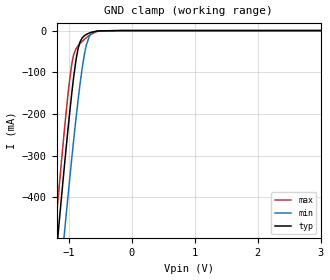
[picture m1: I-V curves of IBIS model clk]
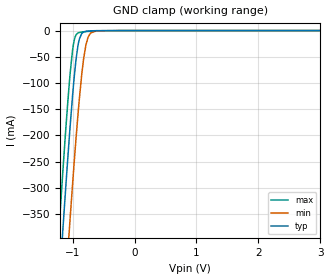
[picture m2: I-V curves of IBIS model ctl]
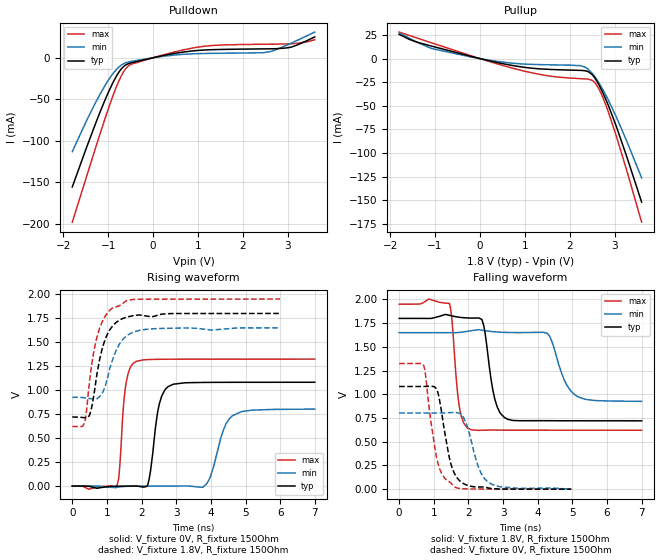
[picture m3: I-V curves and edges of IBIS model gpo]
|Texas Instruments Incorporated
| TPS650860 Configurable Multi-Rail PMIC for 2S & 3S Li-Ion
| Battery-Operated Devices
| Marketing part#   Digital Voltage Range   Package-type   #pins
| TPS650860A0RSKT   1.65V - 1.95V   VQFN   64
[IBIS Ver]   4.1
[File name]   tps650860.ibs
[File Rev]   1.0
[Date]   9/9/2015
[Source]
| Texas Instruments Incorporated.
| Analog-eLab Design Center, HPA
| 12500 TI Blvd
| Dallas, TX -75243
[Notes]   Revision History:
| Rev 1.0: 9/9/2015
| - Initial version of the model
| - Model generated from simulations in TISPICE
| - Model matched to SPICE simulation
| - C_comp although listed in numerical order of value are
|   obtained from varying PVT conditions. For PVT conditions for
|   each specific value refer the buffer description under
|   respective [Model]. IBIS model user is responsible for using
|   appropriate C_comp to simulate for Signal Integrity.
[Disclaimer]
| This model is designed as an aid for customers of Texas Instruments.
| TI and its licensors and suppliers make no warranties, either expressed
| or implied, with respect to this  model, including the warranties of
| merchantability or fitness for a particular purpose. The model is
| provided solely on an "as is" basis. The entire risk as to its quality
| and performance is with the customer.
[Copyright]
(C) Copyright 2014 Texas Instruments Incorporated.All rights reserved.
|   TPS650860A0RSKT
[Component]   TPS650860A0RSKT
[Manufacturer]   TI
[Package]   |64 VQFN  -  RSK package
|   typ   min   max
R_pkg   0.2   0.16   0.24
L_pkg   1.5nH   1.2nH   1.8nH
C_pkg   0.4pF   0.32pF   0.48pF
[Pin]  signal_name   model_name   R_pin   L_pin   C_pin
1   FBGND2   nc   NA   NA   NA
2   FBVOUT2   nc   NA   NA   NA
3   DRVH2   nc   NA   NA   NA
4   SW2   nc   NA   NA   NA
5   BOOT2   nc   NA   NA   NA
6   PGNDSNS2   gnd   NA   NA   NA
7   DRVL2   nc   NA   NA   NA
8   DRV5V_2_A1   power   NA   NA   NA
9   LDOA1   nc   NA   NA   NA
10   LX3   nc   NA   NA   NA
11   PVIN3   power   NA   NA   NA
12   FB3   nc   NA   NA   NA
13   CTL1   ctl   NA   NA   NA
14   CTL6/SLPENB2   ctl   NA   NA   NA
15   IRQB   irqb   NA   NA   NA
16   GPO1   gpox   NA   NA   NA
17   SWB1   nc   NA   NA   NA
18   PVINSWB1_B2   power   NA   NA   NA
19   SWB2   nc   NA   NA   NA
20   LX5   nc   NA   NA   NA
21   PVIN5   power   NA   NA   NA
22   FB5   nc   NA   NA   NA
23   FB4   nc   NA   NA   NA
24   PVIN4   power   NA   NA   NA
25   LX4   nc   NA   NA   NA
26   GPO2   gpox   NA   NA   NA
27   GPO3   gpox   NA   NA   NA
28   GPO4   gpox   NA   NA   NA
29   FBVOUT1   nc   NA   NA   NA
30   ILIM1   nc   NA   NA   NA
31   SWA1   nc   NA   NA   NA
32   PVINSWA1   power   NA   NA   NA
33   DRVH1   nc   NA   NA   NA
34   SW1   nc   NA   NA   NA
35   BOOT1   nc   NA   NA   NA
36   PGNDSNS1   gnd   NA   NA   NA
37   DRVL1   nc   NA   NA   NA
38   DRV5V_1_6   power   NA   NA   NA
39   DRVL6   nc   NA   NA   NA
40   PGNDSNS6   gnd   NA   NA   NA
41   BOOT6   nc   NA   NA   NA
42   SW6   nc   NA   NA   NA
43   DRVH6   nc   NA   NA   NA
44   FBVOUT6   nc   NA   NA   NA
45   ILIM6   nc   NA   NA   NA
46   PVINVTT   power   NA   NA   NA
47   VTT   nc   NA   NA   NA
48   VTTFB   nc   NA   NA   NA
49   LDOA3   nc   NA   NA   NA
50   PVINLDOA2_A3   power   NA   NA   NA
51   LDOA2   nc   NA   NA   NA
52   AGND   gnd   NA   NA   NA
53   VREF   nc   NA   NA   NA
54   LDO3P3   nc   NA   NA   NA
55   VSYS   power   NA   NA   NA
56   LDO5P0   nc   NA   NA   NA
57   V5ANA   power   NA   NA   NA
58   CLK   clk   NA   NA   NA
59   DATA   data   NA   NA   NA
60   CTL2   ctl   NA   NA   NA
61   CTL3/SLPENB1   ctl   NA   NA   NA
62   CTL4   ctl   NA   NA   NA
63   CTL5   ctl   NA   NA   NA
64   ILIM2   nc   NA   NA   NA
|   Model Selectors
[Model Selector] data
data_std   1.8V  digital I/O_Open_drain
data_hs   1.8V  digital I/O_Open_drain
[Model Selector] gpox
gpo   1.8V  digital Output
gpo_od   1.8V  digital Open_drain
| Models and submodels in the file (7): clk (Input), ctl (Input), gpo (Output), gpo_od (Open_drain), data_std (I/O_open_drain), data_hs (I/O_open_drain), irqb (Open_drain)
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|   clk Model
[Model]   clk
Model_type   Input
Vinl = 0.4
Vinh = 1.2
|   typ   min   max
|   (nom PVT)   (fast PVT)   (slow PVT)
C_comp   1.465e-12   1.404e-12   1.531e-12
| Where nom  PVT is Nominal Process, 1.8V, 27C
|   Fast PVT is Strong Process,  1.95V, -40C
|   Slow PVT is Weak Process,   1.65V, 125C
[Voltage Range]   1.8   1.65   1.95
|Junction Temperature
[Temperature Range]   27   125   -40
[Power Clamp Reference]   1.8   1.65   1.95
[GND Clamp Reference]   0   0   0
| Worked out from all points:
|   GND clamp passes 1 mA (typ) near -0.54 V on its own axis
[GND Clamp]
|   Voltage   I(typ)   I(min)   I(max)
-1.8V     -1.585A    -1.712A    -1.529A
-1.417V   -903.9mA   -1.052A    -830.1mA
-1.201V   -532.4mA   -690.5mA   -448.4mA
-1.17V    -480.2mA   -639.5mA   -395mA
-1.076V   -327.4mA   -488.9mA   -240.6mA
-959.6mV  -153.1mA   -309.5mA   -82.58mA
-887.4mV  -67.95mA   -206.8mA   -42.91mA
-828mV    -27.88mA   -130.5mA   -31.56mA
-722.6mV  -8.948mA   -32.89mA   -16.64mA
-648.3mV  -4.138mA   -7.502mA   -8.538mA
-516.9mV  -657.9uA   -778.2uA   -1.114mA
3.6V      0A         0A         0A
[POWER Clamp]
|   Voltage   I(typ)   I(min)   I(max)
-1.8V     0A         0A         0A
0V        0A         0A         0A
3.6V      0A         0A         0A
|   ctl Model
[Model]   ctl
Model_type   Input
Vinl = 0.4
Vinh = 1.2
|   typ   min   max
|   (nom PVT)   (fast PVT)   (slow PVT)
C_comp   4.431e-13   4.006e-13   4.876e-13
| Where nom  PVT is Nominal Process, 1.8V, 27C
|   Fast PVT is Strong Process,  1.95V, -40C
|   Slow PVT is Weak Process,   1.65V, 125C
[Voltage Range]   1.8   1.65   1.95
|Junction Temperature
[Temperature Range]   27   125   -40
[Power Clamp Reference]   1.8   1.65   1.95
[GND Clamp Reference]   0   0   0
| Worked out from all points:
|   GND clamp passes 1 mA (typ) near -0.76 V on its own axis
[GND Clamp]
|   Voltage   I(typ)   I(min)   I(max)
-1.8V     -1.6A      -1.776A    -1.496A
-1.224V   -501.7mA   -684.6mA   -389.4mA
-1.153V   -374.6mA   -556.8mA   -263mA
-1.054V   -206.9mA   -383.9mA   -102.9mA
-986.4mV  -106.2mA   -271.9mA   -26.76mA
-959.6mV  -72.63mA   -229.8mA   -12.55mA
-914.4mV  -30.13mA   -163.2mA   -4.668mA
-851.2mV  -5.575mA   -83.45mA   -2.788mA
-784.8mV  -1.372mA   -27.75mA   -1.943mA
-711mV    -557uA     -4.86mA    -1.184mA
-610.3mV  -144uA     -385.6uA   -415.3uA
3.6V      0A         0A         0A
[POWER Clamp]
|   Voltage   I(typ)   I(min)   I(max)
-1.8V     0A         0A         0A
0V        0A         0A         0A
3.6V      0A         0A         0A
|   gpo Model
[Model]   gpo
Model_type   Output
Polarity   Non-Inverting
Vmeas = 0.9
Vref = 0
Cref = 2pF
Rref = 200
|   typ   min   max
|   (nom PVT)   (fast PVT)   (slow PVT)
C_comp   1.043e-12   7.832e-13   1.236e-12
| Where nom  PVT is Nominal Process, 1.8V, 27C
|   Fast PVT is Strong Process,  1.95V, -40C
|   Slow PVT is Weak Process,   1.65V, 125C
[Voltage Range]   1.8   1.65   1.95
|Junction Temperature
[Temperature Range]   27   125   -40
[Pullup Reference]   1.8   1.65   1.95
[Pulldown Reference]   0   0   0
[Power Clamp Reference]   1.8   1.65   1.95
[GND Clamp Reference]   0   0   0
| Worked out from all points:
|   slope of the pulldown table from 0 to 0.27 V, typ, clamps not added: 86.2 ohm
|   slope of the pullup table from 0 to 0.27 V, typ, clamps not added: 91 ohm
|   falling waveform, V_fixture 1.8V, R_fixture 150Ohm: 20-80 % time 269ps typ, 431ps min, 184ps max; typ from 1.8 V to 0.721 V
|   rising waveform, V_fixture 0V, R_fixture 150Ohm: 20-80 % time 241ps typ, 387ps min, 165ps max; typ from 0 V to 1.08 V
|   rising waveform, V_fixture 1.8V, R_fixture 150Ohm: 20-80 % time 399ps typ, 435ps min, 392ps max; typ from 0.72 V to 1.8 V
|   falling waveform, V_fixture 0V, R_fixture 150Ohm: 20-80 % time 337ps typ, 393ps min, 320ps max; typ from 1.08 V to 0 V
[Pulldown]
|   Voltage   I(typ)   I(min)   I(max)
-1.8V     -155.6mA   -113.1mA   -198mA
-1.314V   -83.91mA   -57.48mA   -114.2mA
-986.4mV  -40.45mA   -26.15mA   -59.81mA
-755.6mV  -16.81mA   -10.72mA   -27.16mA
-649.5mV  -10.19mA   -6.943mA   -16.12mA
-552.6mV  -7.182mA   -5.154mA   -9.916mA
252mV     2.94mA     1.922mA    3.888mA
1.006V    8.834mA    4.97mA     12.84mA
1.472V    9.956mA    5.428mA    15.23mA
2.622V    10.77mA    7.539mA    16.37mA
3.087V    12.98mA    17.87mA    16.83mA
3.6V      25.13mA    30.91mA    21.68mA
[Pullup]
|   Voltage   I(typ)   I(min)   I(max)
-1.8V     25.69mA    27.3mA     28.08mA
-1.077V   13.22mA    10.67mA    16.69mA
-1.8mV    20.64uA    15.02uA    27.04uA
803.3mV   -7.909mA   -5.186mA   -11.07mA
1.512V    -11.33mA   -6.532mA   -18.17mA
2.231V    -12.48mA   -7.467mA   -21.22mA
2.394V    -13.51mA   -10.7mA    -21.69mA
2.522V    -18.21mA   -16.88mA   -23.77mA
2.666V    -29.27mA   -26.99mA   -33.72mA
2.864V    -50.28mA   -44.51mA   -57.31mA
3.256V    -102.1mA   -86.06mA   -116.5mA
3.6V      -151.9mA   -126.3mA   -173.2mA
[Ramp]
R_load = 150
|   typ   min   max
dV/dt_r   0.649427/2.38409e-10   0.48153/3.82364e-10   0.794353/1.64502e-10
dV/dt_f   0.647574/2.66069e-10   0.434522/4.256e-10   0.797069/1.82983e-10
[Falling Waveform]
V_fixture = 1.8V
V_fixture_min = 1.65V
V_fixture_max = 1.95V
R_fixture = 150Ohm
|   Time   V(typ)   V(min)   V(max)
0s        1.8V       1.65V      1.95V
1.452ns   1.833V     1.65V      1.958V
1.718ns   1.813V     1.652V     916.8mV
1.966ns   1.805V     1.664V     646.7mV
2.39ns    1.787V     1.676V     622mV
2.76ns    950.3mV    1.659V     623.3mV
3.036ns   756.5mV    1.653V     622.8mV
4.274ns   722mV      1.643V     622.1mV
5.184ns   721.2mV    970.1mV    621.9mV
6.998ns   720.7mV    925.8mV    621.6mV
[Rising Waveform]
V_fixture = 0V
V_fixture_min = 0V
V_fixture_max = 0V
R_fixture = 150Ohm
|   Time   V(typ)   V(min)   V(max)
0s        542.7pV    23.29nV    169.3pV
1.272ns   -1.556mV   -13.26mV   -8.677mV
1.55ns    -567.4uV   -3.406mV   1.068V
1.856ns   454.5uV    -791.3uV   1.301V
2.17ns    1.338mV    -261.6uV   1.319V
2.51ns    853.6mV    -142.1uV   1.322V
2.768ns   1.037V     -105.4uV   1.323V
3.86ns    1.081V     17.58mV    1.323V
4.628ns   1.082V     734.7mV    1.323V
6.998ns   1.082V     802.5mV    1.324V
[Rising Waveform]
V_fixture = 1.8V
V_fixture_min = 1.65V
V_fixture_max = 1.95V
R_fixture = 150Ohm
|   Time   V(typ)   V(min)   V(max)
0s        720.4mV    925.4mV    621.3mV
336ps     713.6mV    920.9mV    646.7mV
396ps     713.6mV    918.1mV    737.5mV
488ps     731.2mV    913.4mV    1.055V
604ps     907.9mV    908.6mV    1.364V
778ps     1.3V       928.9mV    1.633V
1.172ns   1.672V     1.327V     1.859V
1.458ns   1.747V     1.529V     1.905V
1.942ns   1.784V     1.624V     1.948V
5.998ns   1.8V       1.65V      1.95V
[Falling Waveform]
V_fixture = 0V
V_fixture_min = 0V
V_fixture_max = 0V
R_fixture = 150Ohm
|   Time   V(typ)   V(min)   V(max)
0s        1.083V     803mV      1.324V
714ps     1.083V     803mV      1.297V
1.066ns   1.063V     802.8mV    360.4mV
1.216ns   833.4mV    803mV      174.1mV
1.436ns   353.6mV    806.1mV    80.6mV
1.594ns   167.1mV    809.5mV    27.8mV
1.866ns   57.04mV    750.9mV    4.332mV
2.294ns   22.79mV    225.2mV    1.931mV
2.568ns   13.43mV    75.33mV    1.318mV
4.966ns   457.1uV    1.173mV    452.7uV
